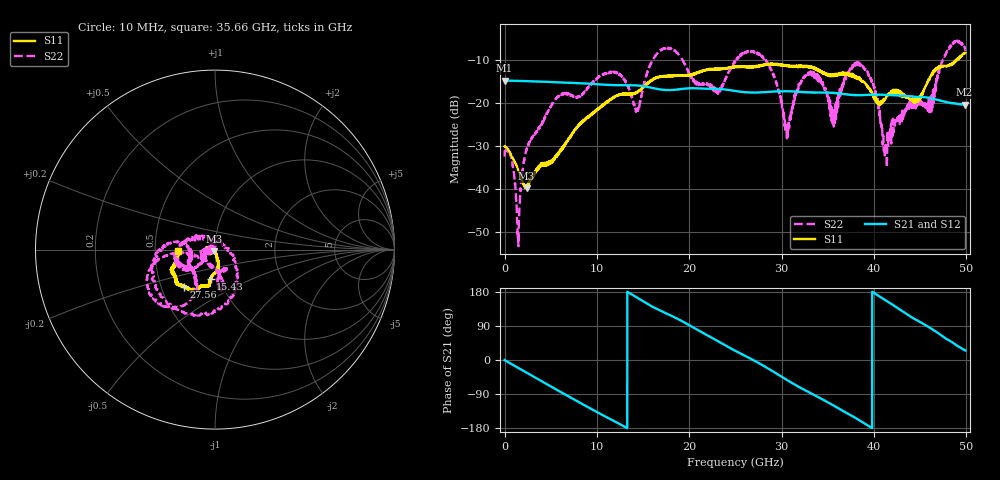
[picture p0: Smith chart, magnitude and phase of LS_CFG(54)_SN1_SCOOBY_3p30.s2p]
!Keysight Technologies,N5245B,MY58422026,A.13.80.08
!Date: Thursday, March 19, 2020 23:43:49
!Correction: S11(Full 2 Port(1,2))
!S21(Full 2 Port(1,2))
!S12(Full 2 Port(1,2))
!S22(Full 2 Port(1,2))
!S2P File: Measurements: S11, S21, S12, S22:
# Hz S DB R 50.0
!freq dBS11 angS11 dBS21 angS21 dBS12 angS12 dBS22 angS22
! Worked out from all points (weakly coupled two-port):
!   4991 points, 10 MHz to 49.91 GHz, reference 50 ohm
!   highest |S21| = -14.75 dB at 10 MHz (marker M1); lowest = -20.4 dB at 49.82 GHz (marker M2)
!   lowest |S11| = -39.8 dB at 2.39 GHz (marker M3), VSWR 1.02, Z = 49.5 - j0.895 ohm
!   |S11| at or under -10 dB: start of sweep to 48.89 GHz; 48.93894 GHz to 48.99009 GHz (51.15 MHz wide, 0.104 % of centre)
!   |S22| runs from -53.3 to -5.4 dB; largest |S21 - S12| = 0.0017
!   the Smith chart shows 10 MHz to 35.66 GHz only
!   S11 on the Smith chart (normalised r, x): 10 MHz: 0.94, -0.01; 15.43 GHz: 0.90, -0.30; 27.56 GHz: 0.65, -0.29; 35.66 GHz: 0.66, -0.01
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1e7  -30.04 -175.0  -14.75 -0.3  -14.74 -0.3  -32.48 177.4
7.8e8  -32.36 -178.6  -14.81 -11.1  -14.80 -11.0  -33.07 -159.1
1.46e9  -35.50 -161.5  -14.84 -20.5  -14.83 -20.5  -51.44 136.4
2.39e9  -39.80 -117.9  -14.90 -33.5  -14.89 -33.5  -30.70 92.8
5.64e9  -32.22 -73.8  -15.16 -78.4  -15.15 -78.4  -18.83 -87.5
8.33e9  -24.71 -75.7  -15.39 -114.9  -15.38 -114.9  -18.13 -73.2
1.204e10  -18.45 -81.6  -15.83 -163.5  -15.83 -163.5  -12.91 -80.7
1.435e10  -17.60 -92.7  -15.90 164.8  -15.90 164.9  -22.31 -127.3
1.543e10  -15.67 -98.5  -16.22 148.9  -16.22 149.0  -13.15 -175.7
1.665e10  -14.01 -99.6  -16.75 132.8  -16.74 132.8  -8.20 -160.9
2.299e10  -12.16 -114.6  -16.69 51.3  -16.69 51.4  -17.63 -166.5
2.496e10  -11.64 -120.9  -17.15 24.6  -17.14 24.7  -10.42 -178.7
2.756e10  -11.40 -130.2  -17.52 -8.6  -17.52 -8.3  -8.77 -101.9
3.062e10  -11.36 -144.6  -17.25 -53.1  -17.25 -52.8  -25.60 59.7
3.328e10  -11.67 -157.7  -17.52 -89.2  -17.51 -88.8  -12.90 -160.2
3.566e10  -13.71 -178.7  -17.62 -120.5  -17.55 -120.0  -25.39 178.7
3.85e10  -14.33 171.6  -18.15 -159.9  -18.13 -160.1  -11.10 -154.7
4.16e10  -17.79 103.5  -18.12 152.4  -18.15 152.3  -26.82 120.9
4.675e10  -11.87 8.1  -19.17 74.6  -19.20 74.7  -14.71 -141.6
4.841e10  -10.97 -6.1  -20.04 47.8  -20.07 47.8  -6.33 -63.0
4.982e10  -8.42 -15.8  -20.38 26.0  -20.39 26.2  -6.95 -11.7
4.991e10  -8.35 -14.9  -20.36 25.0  -20.38 25.0  -7.54 -11.9
